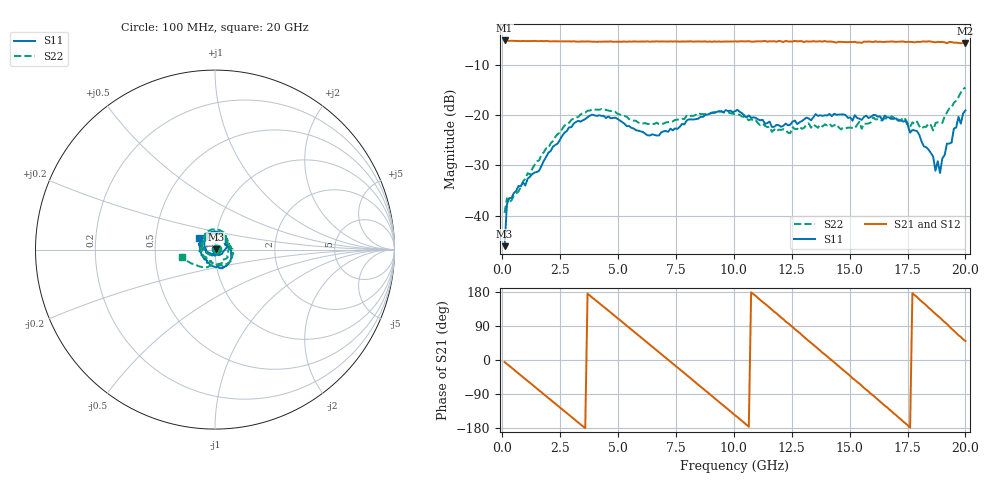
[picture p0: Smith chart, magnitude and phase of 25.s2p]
!Agilent Technologies,N5230C,MY49001569,A.09.33.09
!Agilent N5230C: A.09.33.09
!Date: Tuesday, July 28, 2015 14:52:45
!Correction: S11(Full 2 Port(1,2))
!S21(Full 2 Port(1,2))
!S12(Full 2 Port(1,2))
!S22(Full 2 Port(1,2))
!S2P File: Measurements: S11, S21, S12, S22:
# Hz S  dB  R 50
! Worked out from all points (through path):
!   201 points, 100 MHz to 20 GHz, reference 50 ohm
!   highest |S21| = -5.21 dB at 100 MHz (marker M1); lowest = -5.8 dB at 20 GHz (marker M2)
!   group delay of S21, straight-line fit = 142 ps
!   lowest |S11| = -46.0 dB at 100 MHz (marker M3), VSWR 1.01, Z = 50.4 + j0.299 ohm
!   |S11| at or under -10 dB: start of sweep to end of sweep
!   |S22| runs from -39.4 to -14.5 dB; largest |S21 - S12| = 0.019
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1e8  -46.01 36.3  -5.21 -5.4  -5.20 -5.0  -39.38 17.6
1.995e8  -37.73 11.5  -5.24 -10.6  -5.24 -10.4  -36.52 -3.1
2.99e8  -36.49 -4.1  -5.30 -15.2  -5.26 -15.4  -37.34 -5.5
1.891e9  -28.29 -152.5  -5.30 -95.4  -5.32 -95.4  -26.61 -150.9
3.483e9  -21.04 110.9  -5.40 -174.9  -5.43 -175.3  -19.62 118.9
4.279e9  -20.16 75.7  -5.46 145.1  -5.41 145.4  -18.83 85.2
5.1745e9  -21.38 47.8  -5.47 100.5  -5.41 100.2  -20.08 55.7
5.9705e9  -23.23 34.1  -5.42 60.7  -5.41 60.1  -21.63 38.5
6.7665e9  -24.07 23.8  -5.43 20.5  -5.41 20.1  -21.80 24.3
7.5625e9  -22.75 10.3  -5.41 -19.6  -5.41 -20.2  -20.90 6.6
8.5575e9  -20.36 -18.3  -5.41 -69.9  -5.42 -70.5  -19.79 -14.5
1.005e10  -19.25 -66.6  -5.37 -145.8  -5.45 -146.0  -19.85 -52.5
1.1045e10  -20.89 -104.6  -5.40 163.4  -5.31 162.8  -21.67 -84.6
1.204e10  -22.35 -148.5  -5.38 112.2  -5.42 112.5  -22.95 -122.0
1.3433e10  -20.46 145.8  -5.33 40.8  -5.49 39.9  -21.86 173.2
1.4428e10  -19.93 118.4  -5.62 -10.8  -5.44 -12.2  -21.84 140.6
1.5423e10  -20.73 98.1  -5.60 -62.4  -5.49 -64.3  -21.35 123.8
1.67165e10  -20.48 68.7  -5.45 -130.6  -5.45 -131.1  -20.93 82.7
1.77115e10  -22.97 21.8  -5.52 176.5  -5.47 175.3  -21.45 23.2
1.89055e10  -31.51 -104.9  -5.52 111.4  -5.61 110.0  -21.45 -84.1
1.9204e10  -25.67 -161.0  -5.75 94.9  -5.51 94.0  -19.48 -112.7
2e10  -19.10 143.1  -5.79 50.2  -5.85 48.9  -14.54 -167.3
